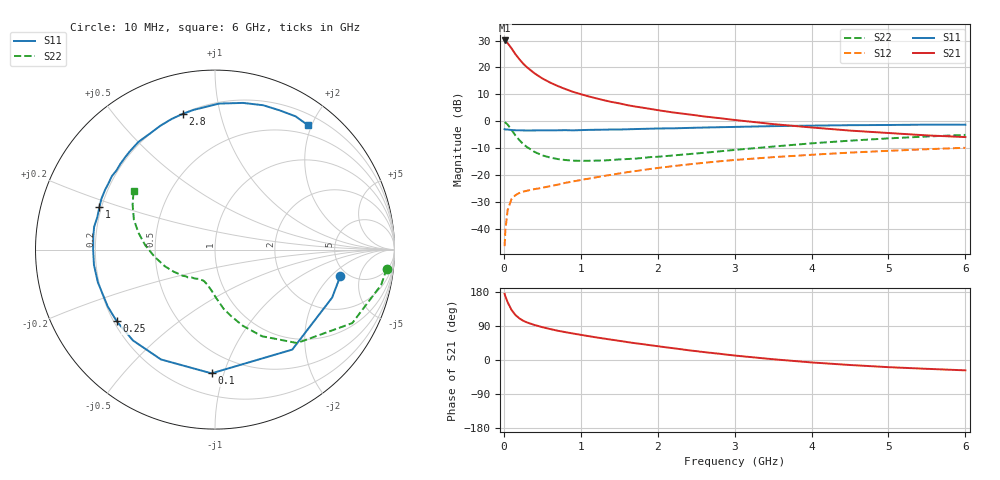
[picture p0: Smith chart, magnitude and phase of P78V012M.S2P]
! SIEMENS Small Signal Semiconductors
! BFP196
! Si NPN RF Bipolar Junction Transistor in SOT143
! VCE = 8 V  IC = 12 mA
! Common Emitter S-Parameters:  May  1996
# GHz  S  MA  R  50
!  f  S11  S21  S12  S22
! GHz  MAG  ANG  MAG  ANG  MAG  ANG  MAG  ANG
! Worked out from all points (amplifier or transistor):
!   36 points, 10 MHz to 6 GHz, reference 50 ohm
!   highest |S21| = 30.0 dB at 10 MHz (marker M1)
!   |S21| within 3 dB of that: start of sweep to 101.7 MHz
!   unconditionally stable (mu >= 1): 862.5 MHz to 3.468 GHz
!   at 250 MHz: K = 0.43, MSG = 23.8 dB, |S12| = -26.1 dB
!   at 1.4 GHz: K = 1.12, MAG = 11.4 dB, |S12| = -19.8 dB
!   at 6 GHz: K = 0.96, MSG = 2.0 dB, |S12| = -9.8 dB
!   S11 on the Smith chart (normalised r, x): 10 MHz: 4.38, -2.61; 100 MHz: 0.35, -0.91; 250 MHz: 0.21, -0.31; 1 GHz: 0.19, +0.17; 2.8 GHz: 0.20, +0.77; 6 GHz: 0.35, +1.94
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0.01  0.7139 -11.8  31.78 174.5  0.0048 83.2  0.9627 -6.3
0.02  0.7052 -22.3  30.79 167.7  0.0096 76.6  0.9466 -12.0
0.05  0.7041 -52.3  28.27 152.1  0.0227 65.6  0.8674 -28.2
0.1  0.6898 -91.6  22.69 132.1  0.036 50.5  0.6929 -48.7
0.15  0.6821 -116.2  17.7 118.9  0.0425 42.6  0.5494 -61.5
0.2  0.6821 -132.1  14.37 110.2  0.0466 38.0  0.4513 -70.0
0.25  0.6778 -144.0  11.84 103.8  0.0494 35.6  0.3799 -76.5
0.3  0.6764 -152.1  10.1 99.2  0.0514 35.3  0.3335 -81.7
0.4  0.6776 -164.4  7.77 92.3  0.0551 35.7  0.2698 -88.6
0.5  0.6798 -172.8  6.261 86.7  0.0582 36.9  0.2333 -94.0
0.6  0.6789 -179.9  5.261 81.8  0.0626 38.8  0.2126 -98.7
0.7  0.6819 173.9  4.534 77.3  0.0666 40.3  0.1992 -102.8
0.8  0.6853 169.4  3.973 73.5  0.0721 41.3  0.1911 -106.3
1  0.6865 159.7  3.193 66.4  0.0814 43.5  0.1846 -111.4
1.1  0.6934 155.8  2.914 63.0  0.0861 44.2  0.1853 -114.4
1.6  0.7113 137.9  2.006 47.5  0.1133 45.1  0.1992 -127.4
2.2  0.7409 119.5  1.462 31.1  0.1473 42.3  0.2324 -141.3
2.8  0.7774 103.4  1.147 16.5  0.1808 37.0  0.2766 -157.0
3.5  0.814 88.3  0.889 2.0  0.2159 29.6  0.3397 -173.4
4.5  0.848 71.5  0.673 -13.2  0.2625 19.0  0.4373 167.5
5.5  0.8675 58.9  0.548 -23.3  0.3034 8.1  0.5227 151.4
6  0.8651 53.3  0.51 -27.3  0.3226 2.1  0.5602 144.1
